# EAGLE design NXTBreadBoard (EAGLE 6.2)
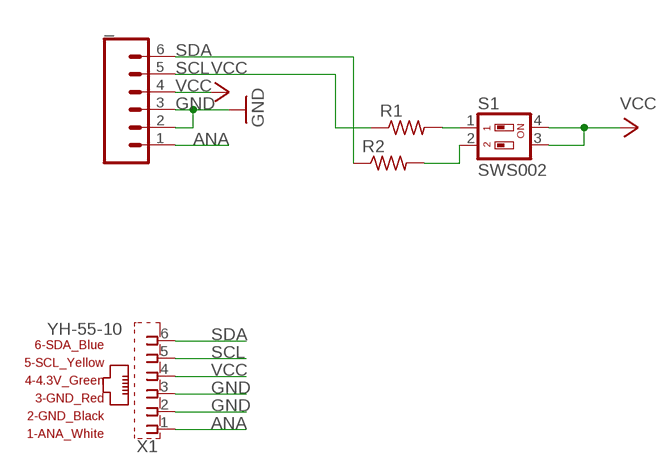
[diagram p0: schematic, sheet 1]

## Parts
_  M06LOCK  [1X06_LOCK]
R1  R-US_M0805  [M0805]
R2  R-US_M0805  [M0805]
S1  SWS002  [SMS-002]
X1  YH-55-10  [YH-55-10]

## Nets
ANA: _.1 X1.1(1_ANA_WHITE)
GND: _.2 _.3 X1.2(2_GND_BLACK) X1.3(3_GND_RED)
N$3: R1.2 S1.1
N$4: R2.2 S1.2
SCL: _.5 R1.1 X1.5(5_SCL_YELLOW)
SDA: _.6 R2.1 X1.6(6_SDA_BLUE)
VCC: _.4 S1.3 S1.4 X1.4(4_4.3V_GREEN)

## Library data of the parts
_ = SparkFun:M06: Header 6 Standard 6-pin 0.1" header. Use with straight break away headers (SKU : PRT-00116), right angle break away headers (PRT-00553), swiss pins (PRT-00743), machine pins (PRT-00117), and female headers (PRT-00115). Molex polarized connector foot print use with SKU : PRT-08094 with associated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
R1 R2 = resistor:R-US_: RESISTOR, American symbol
S1 = smd-special:SWS002: SMD Dip Switch 2 pol.
X1 = DEXTER INDUSTRIES NXT Female Adapter (2!!):YH-55-10: RJ11 6 connects Source:Dexter Industries LEGO MINDSTORMS NXT Female Adapter; OC_FARNELL: unknown; OC_NEWARK: unknown

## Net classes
0 default: width 0.381 mm, drill 0.381 mm, clearance 0.229 mm

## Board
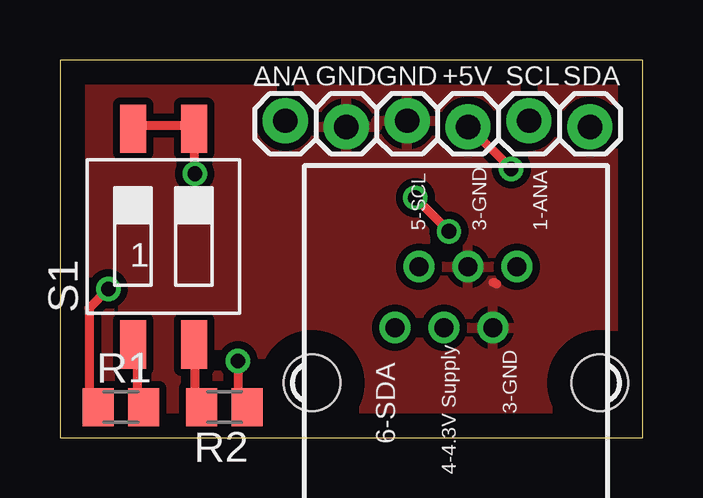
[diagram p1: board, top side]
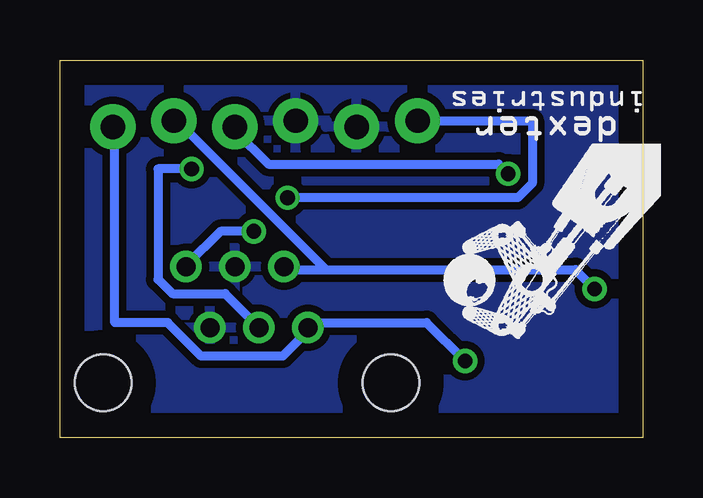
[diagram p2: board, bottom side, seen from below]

Size 24.31 x 15.74 mm. Coordinates in mm from the lower left corner, seen from the top.
Outline: 0,0 24.31,0 24.31,15.74 0,15.74 0,0
Copper layers (1*16): Top 0.035mm / dielectric 1.5mm / Bottom 0.035mm
Design rules: minimum track width 10mil, minimum drill 24mil, track to track 8mil, track to pad 8mil, pad to pad 8mil, via to via 8mil, smd to smd 8mil, copper to edge 40mil, drill to drill 8mil, minimum pad ring 10mil, minimum via ring 8mil, stop-mask expansion 4mil, vias tented up to drill 0mil, thermal gap 10mil

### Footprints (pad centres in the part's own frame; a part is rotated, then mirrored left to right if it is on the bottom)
1X06_LOCK = drill 1.016 pad 1.88: 1 0,0; 2 2.54,-0.254; 3 5.08,0; 4 7.62,-0.254; 5 10.16,0; 6 12.7,-0.254
M0805 = smd 1.3 x 1.6: 1 -0.95,0; 2 0.95,0
SMS-002 = smd 1.092 x 2.007: 1 -1.27,-4.496; 2 1.27,-4.496; 3 1.27,4.496; 4 -1.27,4.496
YH-55-10 = drill 0.8 pad 1.3: 1 2.54,4.84; 2 1.54,2.3; 3 0.5,4.84; 4 -0.5,2.3; 5 -1.54,4.84; 6 -2.54,2.3 | hole 2.36: -6,0; 6,0

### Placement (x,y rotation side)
_  9.4,13.21 0 top
R1  2.54,1.27 0 top
R2  6.86,1.27 180 top
S1  4.32,8.38 0 top
X1  16.51,2.29 0 top

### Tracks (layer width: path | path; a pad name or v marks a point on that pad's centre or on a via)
ANA  (via drill 0.61)
  Top 0.381: v14.82,10 v16.22,8.6
  Bottom 0.381: v16.22,8.6 17.62,8.6 19.02,7.2 X1.1 | v14.82,10 5.22,10 4.62,10.6 4.62,13.2 9.22,13.2 _.1
GND
  Top 0.381: 18.22,6.4 18.07,6.47
  pour Bottom (isolate 0.305): 0.25,15.49 24.13,15.49 24.13,0.25 0.25,0.25
  pour Top (isolate 0.305): 24.13,15.49 24.13,0.25 0.25,0.25 0.25,15.49
N$3
  Top 0.381: R1.2 3.42,1.4 3.22,1.6 3.22,3.8 S1.1
N$4
  Top 0.381: R2.2 5.82,1.4 5.62,1.6 5.62,3.8 S1.2
SCL  (via drill 0.61)
  Top 0.381: v2.02,6.2 1.22,5.4 1.22,1.6 1.42,1.4 R1.1
  Bottom 0.381: v2.02,6.2 2.82,7 13.22,7 | 13.22,7 14.82,7 X1.5 | 13.22,7 19.42,13.2 _.5
SDA  (via drill 0.61)
  Top 0.381: v7.42,3.2 7.42,1.6 7.62,1.4 R2.1
  Bottom 0.381: v7.42,3.2 9.02,4.8 13.62,4.8 13.82,4.6 X1.6 14.02,4.4 15.02,3.4 18.42,3.4 19.82,4.8 22.02,4.8 22.02,12.8 _.6
VCC  (via drill 0.61)
  Top 0.381: S1.4 3.22,13 5.42,13 S1.3 5.62,12.8 v5.62,11 | v18.82,11.2 17.02,13 _.4
  Bottom 0.381: v18.82,11.2 20.22,11.2 20.22,6.6 19.62,6 17.42,6 X1.4 | v5.62,11 6.02,11.4 15.62,11.4 17.02,12.8 _.4

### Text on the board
tNames: ANA | GND | GND | +5V | SCL | SDA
